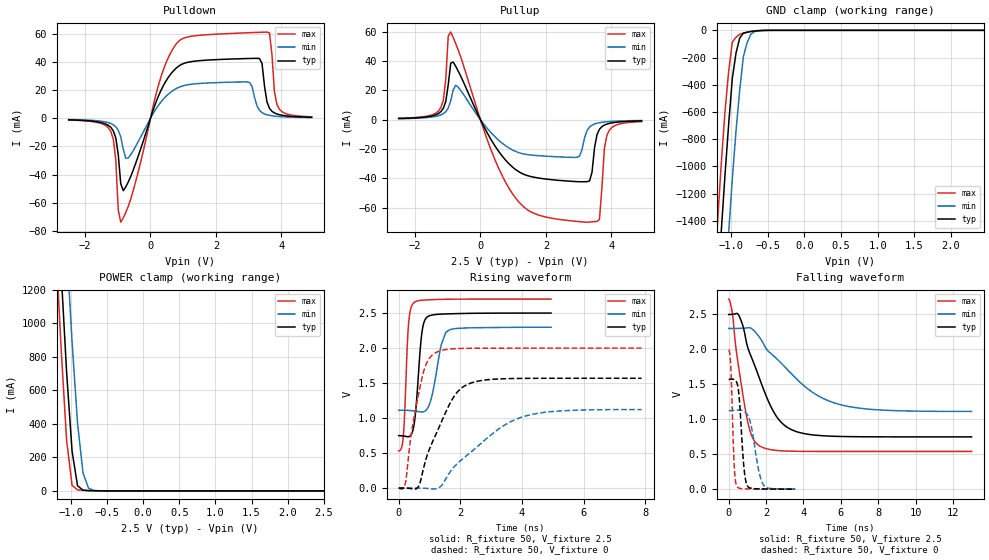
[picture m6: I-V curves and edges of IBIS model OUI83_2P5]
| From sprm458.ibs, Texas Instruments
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|OUI83_2P75; DEFAULT
|   Model Cell OUI83_2P5
|OUI83_2P5
[Model]   OUI83_2P5
Model_type   3-state
Polarity   Non-Inverting
Enable   Active-Low
Cref =  15.0000pF
Rref =  100.000M
Vref =  0V
Vmeas =  1.25
C_comp   1.8698p   1.8104p   1.9947p
[Temperature Range]   25   125   -40
[Voltage Range]   2.5   2.3   2.7
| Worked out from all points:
|   slope of the pulldown table from 0 to 0.375 V, typ, clamps not added: 16.7 ohm
|   slope of the pullup table from 0 to 0.375 V, typ, clamps not added: 24.3 ohm
|   GND clamp passes 1 mA (typ) near -0.57 V on its own axis
|   POWER clamp passes 1 mA (typ) near -0.68 V on its own axis
|   rising waveform, R_fixture 50, V_fixture 2.5: 20-80 % time 183ps typ, 297ps min, 126ps max; typ from 0.749 V to 2.5 V
|   rising waveform, R_fixture 50, V_fixture 0: 20-80 % time 897ps typ, 1.77ns min, 466ps max; typ from 0 V to 1.57 V
|   falling waveform, R_fixture 50, V_fixture 2.5: 20-80 % time 1.51ns typ, 2.8ns min, 720ps max; typ from 2.5 V to 0.748 V
|   falling waveform, R_fixture 50, V_fixture 0: 20-80 % time 236ps typ, 431ps min, 146ps max; typ from 1.57 V to 0.001 V
[POWER_clamp]
|   voltage   I(typ)   I(min)   I(max)
-2.5V     14.33A     15.07A     13.92A
-1.187V   1.745A     2.55A      1.279A
-1.162V   1.527A     2.329A     1.065A
-1.136V   1.31A      2.108A     850.1mA
-1.111V   1.11A      1.897A     667.8mA
-1.061V   710.2mA    1.474A     303.1mA
-1.01V    395mA      1.084A     123.1mA
-984.8mV  237.4mA    889.6mA    33.13mA
-909.1mV  31mA       404mA      6.023mA
-833.3mV  4.304mA    107.2mA    3.736mA
-681.8mV  1.026mA    2.909mA    1.264mA
2.5V      25.45pA    4.321nA    262fA
[Pulldown]
|   voltage   I(typ)   I(min)   I(max)
-2.5V     -1.055mA   -812.8uA   -1.175mA
-1.212V   -6.449mA   -3.675mA   -9.337mA
-1.061V   -13.88mA   -5.986mA   -29.54mA
-909.1mV  -46.47mA   -13.18mA   -73.95mA
-681.8mV  -45.46mA   -28.32mA   -62.79mA
303mV     19mA       11.15mA    28.2mA
984.8mV   38.8mA     23.1mA     56.82mA
3.03V     42.63mA    25.53mA    61mA
3.333V    42.55mA    5.653mA    61.25mA
3.636V    7.153mA    2.123mA    60.83mA
3.864V    3.092mA    1.414mA    10.01mA
4.924V    800.1uA    540.5uA    1.094mA
[Pullup]
|   voltage   I(typ)   I(min)   I(max)
-2.5V     856.4uA    691.1uA    993.4uA
-1.212V   5.468mA    3.266mA    8.205mA
-984.8mV  23.91mA    8.004mA    57.09mA
-909.1mV  38.64mA    12.89mA    59.79mA
-681.8mV  33.25mA    22.23mA    47.64mA
1.061V    -33.75mA   -21.48mA   -53.02mA
2.955V    -42.22mA   -25.6mA    -69.37mA
3.258V    -42.21mA   -7.356mA   -69.88mA
3.636V    -6.5mA     -2.001mA   -68.04mA
3.788V    -3.626mA   -1.52mA    -19.34mA
3.939V    -2.477mA   -1.222mA   -7.104mA
4.924V    -788uA     -530.2uA   -1.239mA
[GND_clamp]
|   voltage   I(typ)   I(min)   I(max)
-2.5V     -14.53A    -15.34A    -14.08A
-1.187V   -1.927A    -2.792A    -1.422A
-1.136V   -1.486A    -2.345A    -988mA
-1.086V   -1.075A    -1.915A    -607.9mA
-1.035V   -698.1mA   -1.498A    -307.7mA
-984.8mV  -355mA     -1.094A    -87.14mA
-934.3mV  -168.4mA   -742.6mA   -51.19mA
-883.8mV  -56.9mA    -442.2mA   -29.15mA
-833.3mV  -20.37mA   -193.1mA   -21.02mA
-782.8mV  -13.75mA   -91.12mA   -14.78mA
-681.8mV  -4.944mA   -9.091mA   -4.753mA
2.449V    23.34pA    119.8nA    217.6fA
[Ramp]
| variable   typ   min   max
dV/dt_f   1.060113/1.510666n   0.7198434/2.810628n   1.30843/0.7200243n
dV/dt_r  0.9501795/0.9004069n  0.6821083/1.781746n   1.208691/0.4668917n
R_load = 50
[Rising Waveform]
R_fixture = 50
V_fixture = 2.5
V_fixture_min = 2.3
V_fixture_max = 2.7
|   time   V(typ)   V(min)   V(max)
0s        749.3mV    1.111V     531.2mV
150ps     744.2mV    1.112V     740mV
324ps     734.1mV    1.11V      2.365V
492ps     885.8mV    1.102V     2.647V
756ps     2.231V     1.087V     2.683V
924ps     2.444V     1.131V     2.688V
1.086ns   2.472V     1.329V     2.692V
1.38ns    2.485V     2.045V     2.696V
1.53ns    2.487V     2.226V     2.697V
4.944ns   2.5V       2.298V     2.7V
[Rising Waveform]
R_fixture = 50
V_fixture = 0
V_fixture_min = 0
V_fixture_max = 0
|   time   V(typ)   V(min)   V(max)
0s        231.9uV    -68.24uV   -3.121mV
228ps     829.3uV    190.8uV    91.17mV
414ps     -8.405mV   425.7uV    786.8mV
642ps     22.25mV    609.7uV    1.334V
912ps     451.5mV    -4.854mV   1.792V
1.194ns   753.8mV    -10.49mV   1.932V
1.8ns     1.312V     303.3mV    1.99V
2.4ns     1.509V     534.7mV    1.997V
4.17ns    1.567V     1.036V     1.999V
7.884ns   1.569V     1.122V     1.999V
[Falling Waveform]
R_fixture = 50
V_fixture = 2.5
V_fixture_min = 2.3
V_fixture_max = 2.7
|   time   V(typ)   V(min)   V(max)
0s        2.499V     2.3V       2.72V
210ps     2.502V     2.299V     2.497V
540ps     2.489V     2.3V       1.735V
1.002ns   2.043V     2.308V     983.3mV
1.284ns   1.843V     2.286V     732.3mV
1.638ns   1.592V     2.178V     621.9mV
2.64ns    1.009V     1.848V     552.3mV
3.78ns    811.2mV    1.539V     541.6mV
6.42ns    752.1mV    1.183V     539.9mV
12.99ns   748.3mV    1.113V     539.9mV
[Falling Waveform]
R_fixture = 50
V_fixture = 0
V_fixture_min = 0
V_fixture_max = 0
|   time   V(typ)   V(min)   V(max)
0s        1.57V      1.124V     1.994V
114ps     1.574V     1.124V     1.751V
300ps     1.569V     1.129V     317.1mV
438ps     1.522V     1.132V     42.02mV
570ps     1.289V     1.132V     12.7mV
810ps     327.3mV    1.115V     4.607mV
1.014ns   41.19mV    1.059V     3.074mV
1.632ns   4.007mV    235.9mV    1.153mV
1.872ns   2.853mV    53.94mV    793.4uV
3.552ns   695.8uV    2.308mV    99.63uV
